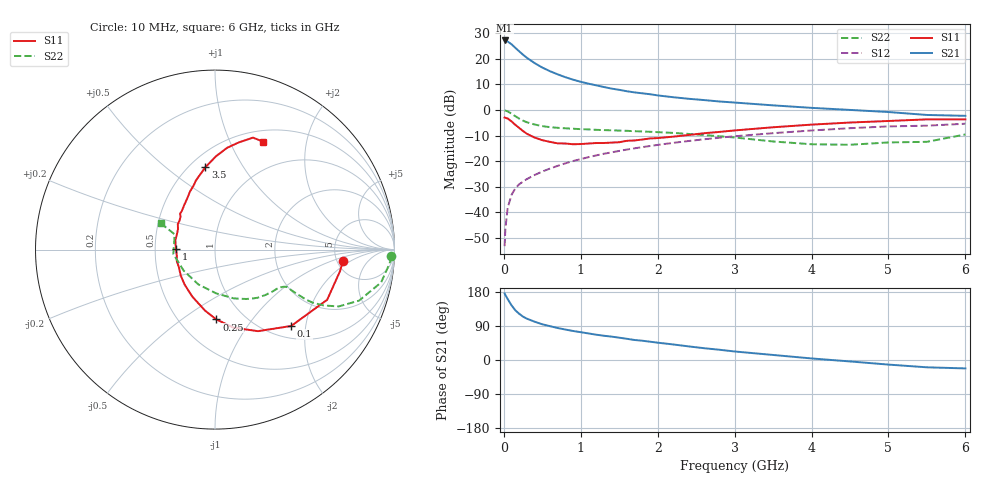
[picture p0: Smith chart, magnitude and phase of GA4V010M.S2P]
! Infineon Technologies  Discrete & RF Semiconductors
! BF775
! Si NPN RF Bipolar Junction Transistor in SOT23
! VCE = 4 V  IC = 10 mA
! Common Emitter S-Parameters:  May  1996
# GHz  S  MA  R  50
!  f  S11  S21  S12  S22
! GHz  MAG  ANG  MAG  ANG  MAG  ANG  MAG  ANG
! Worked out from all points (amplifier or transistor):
!   36 points, 10 MHz to 6 GHz, reference 50 ohm
!   highest |S21| = 27.2 dB at 10 MHz (marker M1)
!   |S21| within 3 dB of that: start of sweep to 153.9 MHz
!   unconditionally stable (mu >= 1): 580.3 MHz to 3.158 GHz
!   at 250 MHz: K = 0.68, MSG = 24.8 dB, |S12| = -27.9 dB
!   at 1.4 GHz: K = 1.11, MAG = 10.4 dB, |S12| = -16.5 dB
!   at 6 GHz: K = 0.94, MSG = 1.5 dB, |S12| = -5.3 dB
!   S11 on the Smith chart (normalised r, x): 10 MHz: 5.66, -1.45; 100 MHz: 1.25, -1.66; 250 MHz: 0.75, -0.68; 1 GHz: 0.64, +0.01; 3.5 GHz: 0.60, +0.69; 6 GHz: 0.63, +1.34
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0.01  0.7158 -5.0  22.88 175.8  0.0022 85.2  0.984 -2.2
0.02  0.7068 -9.8  22.64 171.6  0.0048 84.0  0.9756 -4.6
0.05  0.6847 -24.1  21.79 160.6  0.0124 78.8  0.9433 -11.2
0.1  0.6008 -45.1  19.27 144.3  0.0221 71.0  0.8515 -19.5
0.15  0.5134 -62.3  16.4 131.0  0.0298 65.3  0.7581 -24.7
0.2  0.4474 -76.5  14.02 121.9  0.0356 62.9  0.6806 -27.2
0.25  0.3892 -88.9  12.04 114.4  0.0402 62.0  0.6199 -28.5
0.3  0.3444 -99.3  10.48 109.0  0.045 62.3  0.578 -28.8
0.4  0.2906 -115.9  8.269 101.1  0.054 62.3  0.5229 -28.4
0.5  0.2581 -131.0  6.764 94.2  0.063 63.7  0.4861 -28.1
0.6  0.2396 -142.6  5.739 89.2  0.0722 64.4  0.4639 -27.5
0.7  0.2239 -154.2  4.986 84.4  0.0815 65.0  0.4504 -27.5
0.8  0.2223 -163.3  4.384 80.4  0.0912 64.8  0.4405 -28.0
1  0.2172 178.7  3.564 73.4  0.1102 64.6  0.4244 -29.5
1.1  0.2222 172.2  3.281 70.1  0.1204 64.4  0.4194 -30.8
1.6  0.2513 145.5  2.33 55.9  0.1695 61.2  0.3935 -37.1
2.2  0.3025 124.4  1.784 41.1  0.2289 55.7  0.3584 -48.4
2.8  0.3742 108.8  1.473 27.1  0.2883 49.1  0.3083 -62.7
3.5  0.4617 96.7  1.236 13.3  0.3539 40.4  0.2438 -88.5
4.5  0.5713 83.2  1.007 -3.8  0.443 27.5  0.2102 -146.2
5.5  0.6586 71.3  0.803 -19.3  0.4958 12.6  0.24 159.3
6  0.6582 66.2  0.772 -22.2  0.5416 8.6  0.3341 154.1
